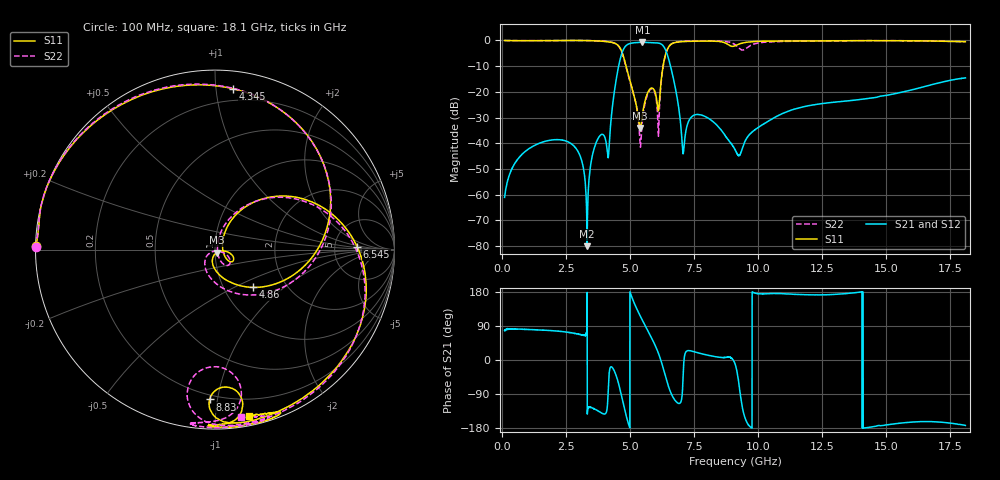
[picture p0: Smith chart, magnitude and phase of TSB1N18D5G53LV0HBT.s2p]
! TSB1N18D5G53LV0HBT  S-PARAMETER MODEL  ( General Type )
! Model Generated by TAIYO YUDEN Corporation (https://www.yuden.co.jp/en/)
! Version 1.0
! TAIYO YUDEN Control No. 190110
! Copyright(c) 2019 TAIYO YUDEN CO.,LTD. All Rights Reserved.
! Products Name : Multilayer Ceramic Devices
! Characteristics :
!  Passband freq : 5150-5925MHz ( At Passband , Insertion Loss : 1.5dB , VSWR 2.0 ),
!  Attenuation : 28dB min at 3300-4200MHz , 20dB min at 7200-7800MHz , Impedance : 50 Ohm ,
!  Case Size : 1.6 x 0.8 / 0.063 x 0.031 [mm/inch] , Thickness : 0.65 / 0.026 [mm/inch]
!  (Conditions: Temperature = 25 degC , DC Bias Current/Voltage = 0A / 0V)
! External Node Assignments :
!  1  o---|-------|---o  2
!  |  BPF  |
! GND o---|-------|---o GND
! Frequency Range : 100MHz  -  18.1GHz  [ 3601 STEP ]
# MHZ S RI R 50
! Freq[MHz].  S11 Real  S11 Imag  S21 Real  S21 Imag  S12 Real  S12 Imag  S22 Real  S22 Imag
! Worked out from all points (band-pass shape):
!   3601 points, 100 MHz to 18.1 GHz, reference 50 ohm
!   highest |S21| = -0.74 dB at 5.485 GHz (marker M1); lowest = -80.0 dB at 3.32 GHz (marker M2)
!   |S21| within 3 dB of the highest: 4.729 GHz to 6.389 GHz (1.661 GHz wide, 29.9 % of centre)
!   lowest |S11| = -34.1 dB at 5.395 GHz (marker M3), VSWR 1.04, Z = 51 - j1.75 ohm
!   |S11| at or under -10 dB: 4.847 GHz to 6.29 GHz (1.444 GHz wide, 25.9 % of centre)
!   |S22| runs from -41.5 to 0.0 dB; largest |S21 - S12| = 0.0023
!   S11 on the Smith chart (normalised r, x): 100 MHz: 0.00, +0.01; 4.345 GHz: 0.12, +1.11; 4.86 GHz: 1.37, -0.63; 6.545 GHz: 8.59, +0.68; 8.83 GHz: 0.17, -0.95; 18.1 GHz: 0.07, -1.23
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100  -0.9973 0.0179  0.00018 0.000869  0.00017 0.000873  -0.9985 0.0171
1385  -0.9815 0.1334  0.00178 0.00954  0.00178 0.00952  -0.9817 0.1364
3100  -0.9222 0.3826  0.00191 0.00439  0.00193 0.00437  -0.9287 0.3699
3320  -0.882 0.4611  -4.87e-05 8.72e-05  -4.46e-05 0.000119  -0.893 0.4448
3690  -0.7463 0.6392  -0.00717 -0.008  -0.00716 -0.00801  -0.7698 0.6191
4150  -0.2906 0.8954  0.0013 -0.00517  0.00134 -0.00511  -0.3286 0.8906
4345  0.1013 0.8958  0.0652 -0.0283  0.0652 -0.028  0.0765 0.9041
4605  0.6412 0.3277  0.0951 -0.4026  0.0963 -0.4024  0.6467 0.2938
4860  0.2115 -0.2105  -0.6989 -0.4016  -0.6986 -0.4024  0.1376 -0.2476
5395  0.00978 -0.0172  -0.4086 0.8215  -0.4096 0.8203  -0.00278 -0.00899
5485  0.0354 -0.00778  -0.2292 0.8898  -0.2306 0.8884  0.0262 -0.0102
5795  0.1041 -0.0509  0.3948 0.8209  0.3929 0.8212  0.0843 -0.0733
6100  0.0431 0.000807  0.8413 0.294  0.8408 0.2946  0.0144 -0.00937
6355  0.355 0.2979  0.5718 -0.4147  0.5713 -0.4145  0.3522 0.292
6545  0.7926 0.0147  0.0763 -0.3652  0.0758 -0.3648  0.7936 -0.016
7080  0.5956 -0.7426  0.00534 -0.00342  0.00534 -0.0034  0.5638 -0.7814
7620  0.3185 -0.9156  0.0343 0.0123  0.0342 0.0121  0.2762 -0.9408
8830  -0.0302 -0.835  0.0117 0.00158  0.0115 0.00159  -0.0905 -0.9339
9100  0.1084 -0.78  0.00748 -0.00125  0.00767 -0.00123  -0.1549 -0.818
12100  -0.0312 -0.9777  -0.0546 0.00778  -0.0548 0.00763  -0.1243 -0.967
15100  0.2399 -0.9644  -0.0861 -0.0143  -0.0861 -0.0147  0.1589 -0.9799
18100  0.1917 -0.9291  -0.1859 -0.0238  -0.185 -0.0239  0.147 -0.9314
